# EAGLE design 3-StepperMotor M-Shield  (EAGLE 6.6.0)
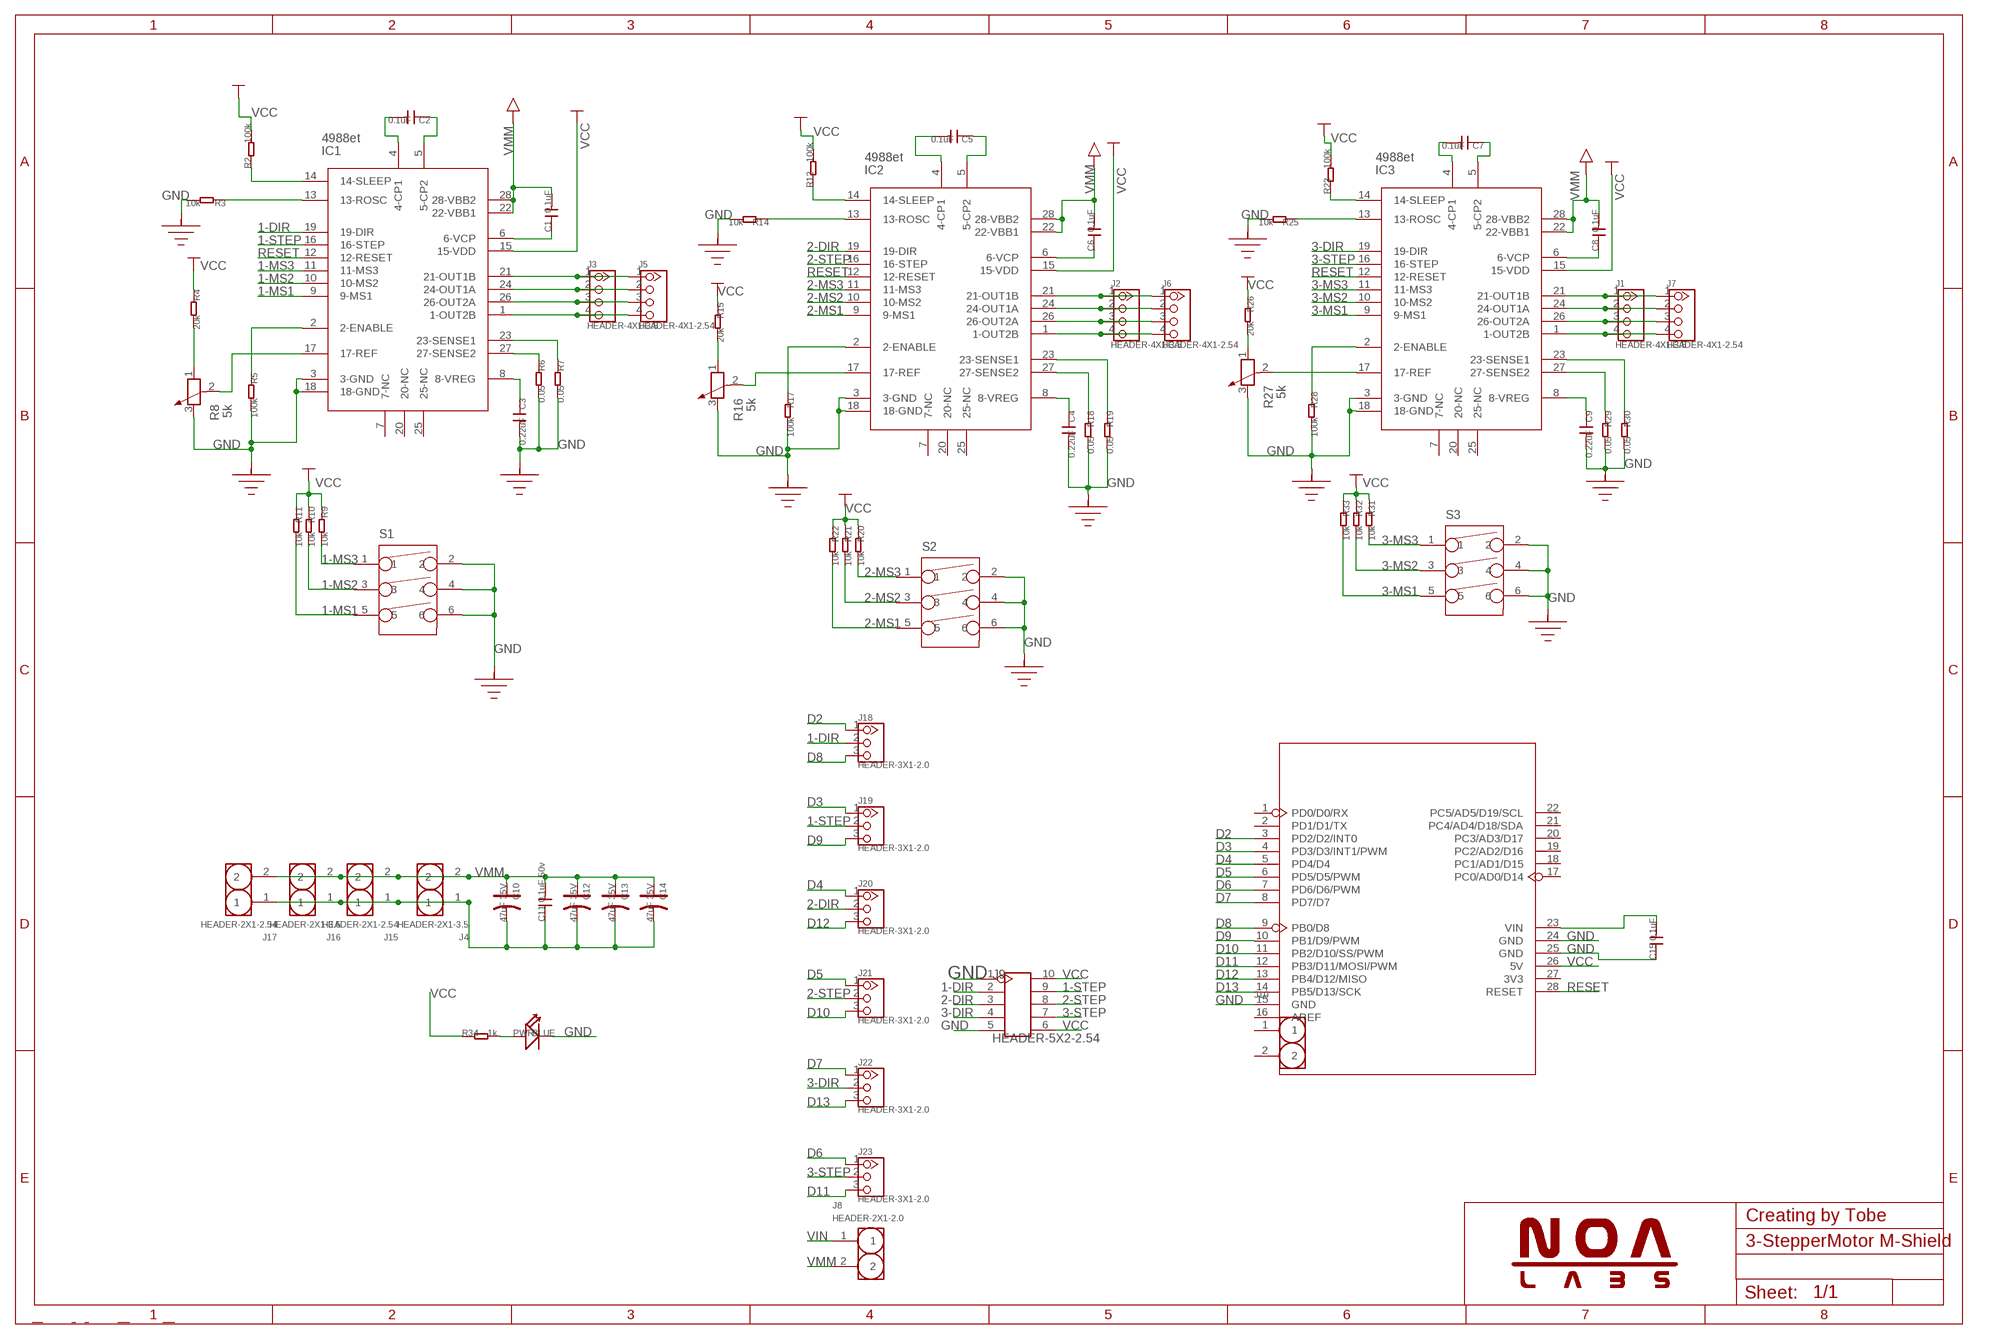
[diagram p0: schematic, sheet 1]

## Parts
C1  0.1uF  C-0603  [0603]
C2  0.1uF  C-0603  [0603]
C3  0.22uF  C-0603  [0603]
C4  0.22uF  C-0603  [0603]
C5  0.1uF  C-0603  [0603]
C6  0.1uF  C-0603  [0603]
C7  0.1uF  C-0603  [0603]
C8  0.1uF  C-0603  [0603]
C9  0.22uF  C-0603  [0603]
C10  47uF 35V  CAP-ELECTRO-E  [ELECTRO-SMD-E-7.8MM]
C11  0.1uF 50v  C-0603  [0603]
C12  47uF 35V  CAP-ELECTRO-E  [ELECTRO-SMD-E-7.8MM]
C13  47uF 35V  CAP-ELECTRO-E  [ELECTRO-SMD-E-7.8MM]
C14  47uF 35V  CAP-ELECTRO-E  [ELECTRO-SMD-E-7.8MM]
C15  0.1uF  C-0603  [0603]
IC1  4988et  A4988Q  [QFN28]
IC2  4988et  A4988Q  [QFN28]
IC3  4988et  A4988Q  [QFN28]
J1  HEADER-4X1-3.5  HEADER-4P3.5  [4P-3.5]
J2  HEADER-4X1-3.5  HEADER-4P3.5  [4P-3.5]
J3  HEADER-4X1-3.5  HEADER-4P3.5  [4P-3.5]
J4  HEADER-2X1-3.5  HEADER-2P3.5  [2P-3.5]
J5  HEADER-4X1-2.54  HEADER-4P-80/40MIL  [4P-2.54-80/40MIL]
J6  HEADER-4X1-2.54  HEADER-4P-80/40MIL  [4P-2.54-80/40MIL]
J7  HEADER-4X1-2.54  HEADER-4P-80/40MIL  [4P-2.54-80/40MIL]
J8  HEADER-2X1-2.0  HEADER-2P-2.0  [2P-2.0]
J9  HEADER-5X2-2.54  HEADER-2X5P-2.54  [2X5P-2.54]
J10  HEADER-2P-65/35MIL  [2P-2.54-65/35MIL]
J15  HEADER-2X1-2.54  HEADER-2P-65/35MIL  [2P-2.54-65/35MIL]
J16  HEADER-2X1-3.5  HEADER-2P3.5  [2P-3.5]
J17  HEADER-2X1-2.54  HEADER-2P-65/35MIL  [2P-2.54-65/35MIL]
J18  HEADER-3X1-2.0  HEADER-3P-2.0  [3P-2.0]
J19  HEADER-3X1-2.0  HEADER-3P-2.0  [3P-2.0]
J20  HEADER-3X1-2.0  HEADER-3P-2.0  [3P-2.0]
J21  HEADER-3X1-2.0  HEADER-3P-2.0  [3P-2.0]
J22  HEADER-3X1-2.0  HEADER-3P-2.0  [3P-2.0]
J23  HEADER-3X1-2.0  HEADER-3P-2.0  [3P-2.0]
PWR  BLUE  LED'0603'  [LED-0603]
R2  100k  R-0603  [0603]
R3  10k  R-0603  [0603]
R4  20k  R-0603  [0603]
R5  100k  R-0603  [0603]
R6  0.05  R-0603  [0603]
R7  0.05  R-0603  [0603]
R8  5k  R-POTENTIOMETER  [3314J]
R9  10k  R-0603  [0603]
R10  10k  R-0603  [0603]
R11  10k  R-0603  [0603]
R12  100k  R-0603  [0603]
R14  10k  R-0603  [0603]
R15  20k  R-0603  [0603]
R16  5k  R-POTENTIOMETER  [3314J]
R17  100k  R-0603  [0603]
R18  0.05  R-0603  [0603]
R19  0.05  R-0603  [0603]
R20  10k  R-0603  [0603]
R21  10k  R-0603  [0603]
R22  10k  R-0603  [0603]
R23  100k  R-0603  [0603]
R25  10k  R-0603  [0603]
R26  20k  R-0603  [0603]
R27  5k  R-POTENTIOMETER  [3314J]
R28  100k  R-0603  [0603]
R29  0.05  R-0603  [0603]
R30  0.05  R-0603  [0603]
R31  10k  R-0603  [0603]
R32  10k  R-0603  [0603]
R33  10k  R-0603  [0603]
R34  1k  R-0603  [0603]
S1  dial switch  DIP-SWITCH-3  [DIP-SWITCH-3]
S2  dial switch  DIP-SWITCH-3  [DIP-SWITCH-3]
S3  dial switch  DIP-SWITCH-3  [DIP-SWITCH-3]
U1  SEEEDUINO-W/O-ISP-HOLE  [SEEEDUINO-W/O-ISP]

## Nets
1-DIR: IC1.19(19-DIR) J9.2 J18.2
1-MS1: IC1.9(9-MS1) R11.2 S1.5
1-MS2: IC1.10(10-MS2) R10.2 S1.3
1-MS3: IC1.11(11-MS3) R9.2 S1.1
1-STEP: IC1.16(16-STEP) J9.9 J19.2
2-DIR: IC2.19(19-DIR) J9.3 J20.2
2-MS1: IC2.9(9-MS1) R22.2 S2.5
2-MS2: IC2.10(10-MS2) R21.2 S2.3
2-MS3: IC2.11(11-MS3) R20.2 S2.1
2-STEP: IC2.16(16-STEP) J9.8 J21.2
3-DIR: IC3.19(19-DIR) J9.4 J22.2
3-MS1: IC3.9(9-MS1) R33.2 S3.5
3-MS2: IC3.10(10-MS2) R32.2 S3.3
3-MS3: IC3.11(11-MS3) R31.2 S3.1
3-STEP: IC3.16(16-STEP) J9.7 J23.2
D2: J18.1 U1.3(PD2/D2/INT0)
D3: J19.1 U1.4(PD3/D3/INT1/PWM)
D4: J20.1 U1.5(PD4/D4)
D5: J21.1 U1.6(PD5/D5/PWM)
D6: J23.1 U1.7(PD6/D6/PWM)
D7: J22.1 U1.8(PD7/D7)
D8: J18.3 U1.9(PB0/D8)
D9: J19.3 U1.10(PB1/D9/PWM)
D10: J21.3 U1.11(PB2/D10/SS/PWM)
D11: J23.3 U1.12(PB3/D11/MOSI/PWM)
D12: J20.3 U1.13(PB4/D12/MISO)
D13: J22.3 U1.14(PB5/D13/SCK)
GND: C3.2 C4.2 C9.2 C10.- C11.1 C12.- C13.- C14.- C15.1 IC1.3(3-GND) IC1.18(18-GND) IC2.3(3-GND) IC2.18(18-GND) IC3.3(3-GND) IC3.18(18-GND) J4.1 J9.1 J9.5 J15.1 J16.1 J17.1 PWR.- R3.2 R5.2 R6.2 R7.2 R8.3 R14.2 R16.3 R17.2 R18.2 R19.2 R25.2 R27.3 R28.2 R29.2 R30.2 S1.2 S1.4 S1.6 S2.2 S2.4 S2.6 S3.2 S3.4 S3.6 U1.15(GND) U1.24(GND) U1.25(GND) ; supply symbol labelled GND_POWER
N$1: IC1.14(14-SLEEP) R2.1
N$2: IC1.17(17-REF) R8.2
N$3: IC2.14(14-SLEEP) R12.1
N$4: IC1.13(13-ROSC) R3.1
N$5: IC1.2(2-ENABLE) R5.1
N$6: IC1.27(27-SENSE2) R6.1
N$7: IC1.23(23-SENSE1) R7.1
N$8: C3.1 IC1.8(8-VREG)
N$9: C1.1 IC1.6(6-VCP)
N$10: IC2.13(13-ROSC) R14.1
N$11: IC3.14(14-SLEEP) R23.1
N$12: C2.1 IC1.5(5-CP2)
N$13: C2.2 IC1.4(4-CP1)
N$14: IC3.13(13-ROSC) R25.1
N$15: IC1.21(21-OUT1B) J3.1 J5.1
N$16: IC1.24(24-OUT1A) J3.2 J5.2
N$17: IC1.26(26-OUT2A) J3.3 J5.3
N$18: IC1.1(1-OUT2B) J3.4 J5.4
N$19: IC2.17(17-REF) R16.2
N$20: R4.2 R8.1
N$21: R15.2 R16.1
N$22: PWR.+ R34.2
N$23: R26.2 R27.1
N$28: IC2.2(2-ENABLE) R17.1
N$30: IC2.27(27-SENSE2) R18.1
N$31: C4.1 IC2.8(8-VREG)
N$32: IC2.23(23-SENSE1) R19.1
N$34: IC2.1(1-OUT2B) J2.4 J6.4
N$35: IC2.26(26-OUT2A) J2.3 J6.3
N$36: IC2.24(24-OUT1A) J2.2 J6.2
N$37: IC2.21(21-OUT1B) J2.1 J6.1
N$38: C6.1 IC2.6(6-VCP)
N$39: IC3.2(2-ENABLE) R28.1
N$40: IC3.17(17-REF) R27.2
N$41: C5.1 IC2.5(5-CP2)
N$42: C5.2 IC2.4(4-CP1)
N$45: C9.1 IC3.8(8-VREG)
N$46: IC3.27(27-SENSE2) R29.1
N$47: IC3.23(23-SENSE1) R30.1
N$48: C8.1 IC3.6(6-VCP)
N$50: C7.1 IC3.5(5-CP2)
N$51: C7.2 IC3.4(4-CP1)
N$59: IC3.21(21-OUT1B) J1.1 J7.1
N$60: IC3.24(24-OUT1A) J1.2 J7.2
N$61: IC3.26(26-OUT2A) J1.3 J7.3
N$62: IC3.1(1-OUT2B) J1.4 J7.4
RESET: IC1.12(12-RESET) IC2.12(12-RESET) IC3.12(12-RESET) U1.28(RESET)
VCC: IC1.15(15-VDD) IC2.15(15-VDD) IC3.15(15-VDD) J9.6 J9.10 R2.2 R4.1 R9.1 R10.1 R11.1 R12.2 R15.1 R20.1 R21.1 R22.1 R23.2 R26.1 R31.1 R32.1 R33.1 R34.1 U1.26(5V) ; supply symbol labelled POWER_BAR
VIN: C15.2 J8.1 U1.23(VIN)
VMM: C1.2 C6.2 C8.2 C10.+ C11.2 C12.+ C13.+ C14.+ IC1.22(22-VBB1) IC1.28(28-VBB2) IC2.22(22-VBB1) IC2.28(28-VBB2) IC3.22(22-VBB1) IC3.28(28-VBB2) J4.2 J8.2 J15.2 J16.2 J17.2 ; supply symbol labelled POWER_ARROW
Unconnected: IC1.7(7-NC) IC1.20(20-NC) IC1.25(25-NC) IC2.7(7-NC) IC2.20(20-NC) IC2.25(25-NC) IC3.7(7-NC) IC3.20(20-NC) IC3.25(25-NC) J10.1 J10.2 U1.1(PD0/D0/RX) U1.2(PD1/D1/TX) U1.16(AREF) U1.17(PC0/AD0/D14) U1.18(PC1/AD1/D15) U1.19(PC2/AD2/D16) U1.20(PC3/AD3/D17) U1.21(PC4/AD4/D18/SDA) U1.22(PC5/AD5/D19/SCL) U1.27(3V3)

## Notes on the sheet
- Creating by Tobe

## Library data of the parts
C1-C9 C11 C15 = Discrete:C*: Ceramic Capacitors
C10 C12-C14 = Discrete:CAP*: Electrolytic Capacitors,Tantalum Capacitors and Super Capacitors
IC1-IC3 = IC:A4988
J1-J3 J5-J7 = Connector:HEADER-4P
J4 J8 J10 J15-J17 = Connector:HEADER-2P
J9 = Connector:HEADER-2X5P
J18-J23 = Connector:HEADER-3P
PWR = Discrete:LED*
R2-R7 R9-R12 R14 R15 R17-R23 R25 R26 R28-R34 = Discrete:R*
R8 R16 R27 = Discrete:R-POTENTIOMETER*: Potentiometer
S1-S3 = Discrete:DIP-SWITCH-3
U1 = Module:SEEEDUINO-W/O-ISP

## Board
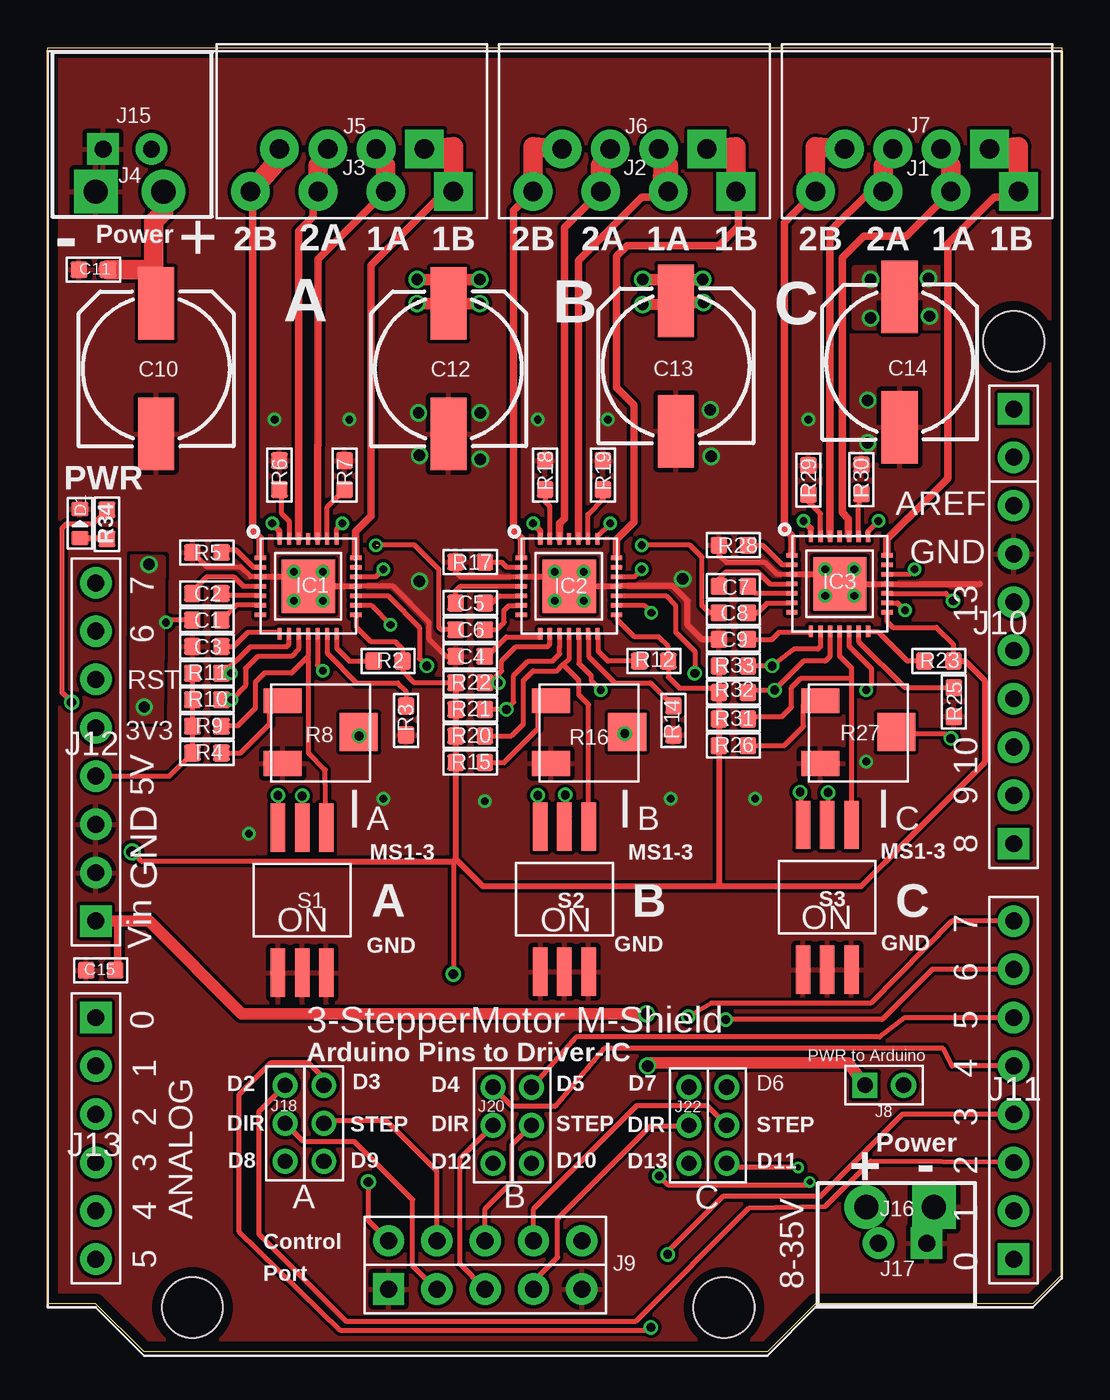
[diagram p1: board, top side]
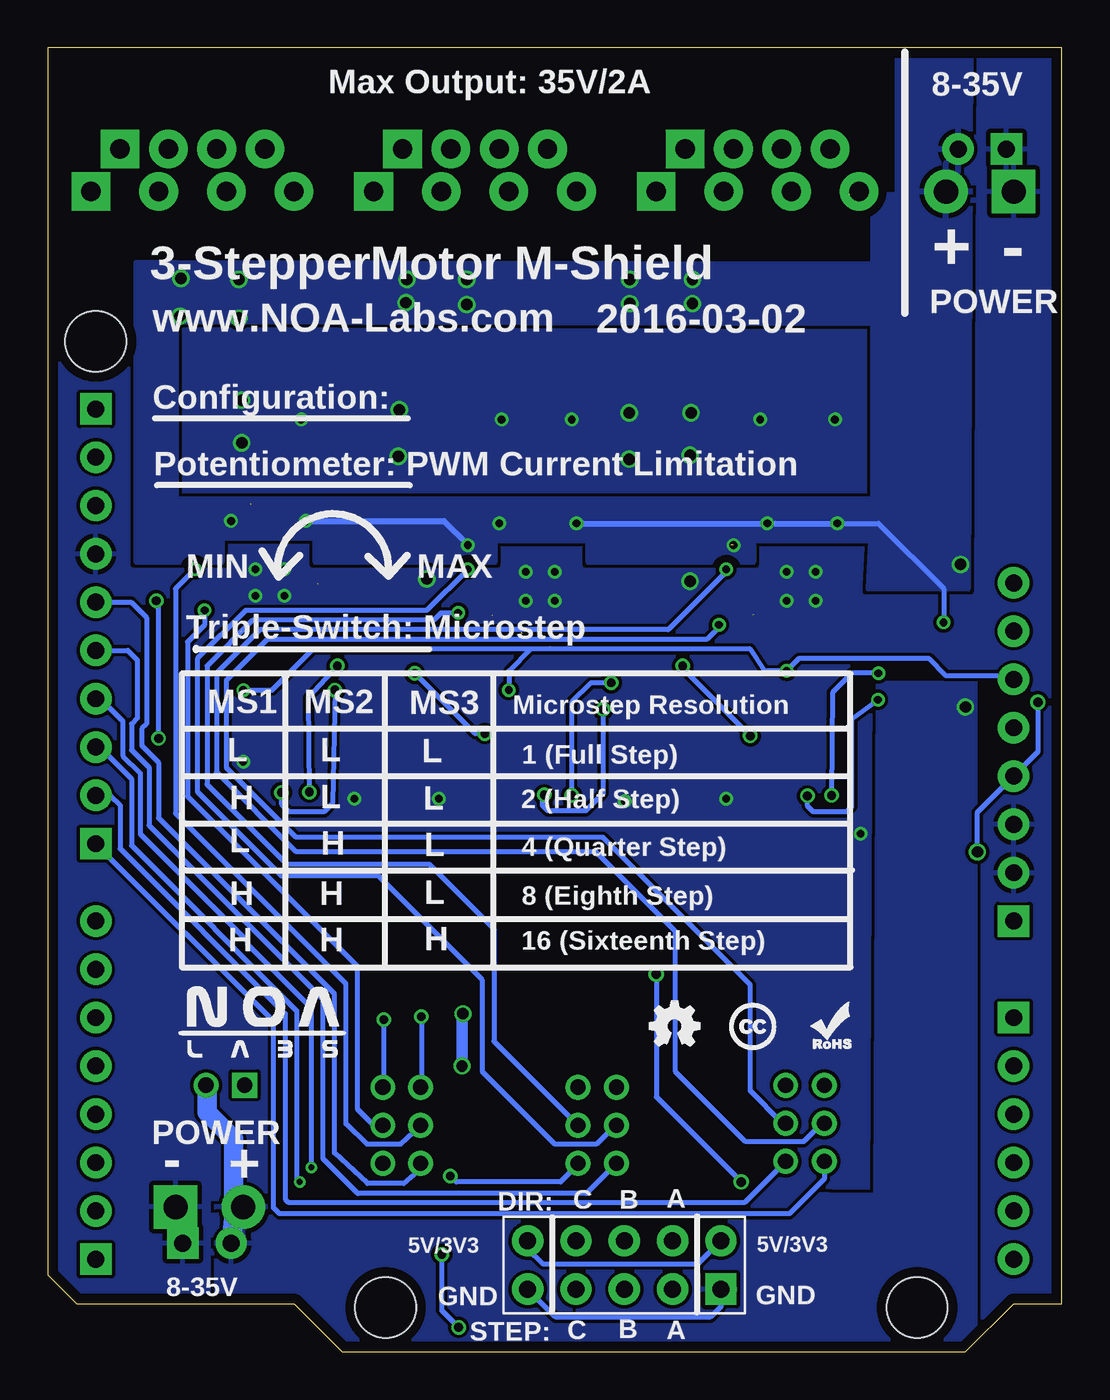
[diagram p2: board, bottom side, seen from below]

Size 53.34 x 68.58 mm. Coordinates in mm from the lower left corner, seen from the top.
Outline: 0,68.58 53.34,68.58 53.34,4.06 51.82,2.54 40.39,2.54 37.85,0 5.08,0 2.54,2.54 0,2.54 0,68.58
Copper layers (1*16): Top 0.035mm / dielectric 1.5mm / Bottom 0.035mm
Design rules "NOA Eagle Rule": minimum track width 7mil, minimum drill 12mil, track to track 7mil, track to pad 7mil, pad to pad 7mil, via to via 7mil, smd to smd 0mil, copper to edge 20mil, drill to drill 10mil, minimum pad ring 10mil, minimum via ring 6mil, stop-mask expansion 2mil, vias tented up to drill 25mil, thermal gap 10mil

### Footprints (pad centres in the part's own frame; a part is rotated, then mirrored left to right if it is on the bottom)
0603 = smd 0.889 x 0.889: 1 -0.762,0; 2 0.762,0
ELECTRO-SMD-E-7.8MM = smd 3.81 x 1.905: + 3.429,0; - -3.429,0
QFN28 = smd 0.6 x 0.23: 1 -2.516,1.5; 2 -2.516,1; 3 -2.516,0.5; 4 -2.516,0; 5 -2.516,-0.5; 6 -2.516,-1; 7 -2.516,-1.5; 15 2.484,-1.5; 16 2.484,-1; 17 2.484,-0.5; 18 2.484,0; 19 2.484,0.5; 20 2.484,1; 21 2.484,1.5 | smd 0.23 x 0.6: 8 -1.516,-2.5; 9 -1.016,-2.5; 10 -0.516,-2.5; 11 -0.016,-2.5; 12 0.484,-2.5; 13 0.984,-2.5; 14 1.484,-2.5; 22 1.484,2.5; 23 0.984,2.5; 24 0.484,2.5; 25 -0.016,2.5; 26 -0.516,2.5; 27 -1.016,2.5; 28 -1.516,2.5 | smd 2.8 x 2.8: 29 0,0
4P-3.5 = drill 1.016 pad 2.032 square: 1 0,5.334 | drill 1.016 pad 2.032: 2 0,1.778; 3 0,-1.778; 4 0,-5.334
2P-3.5 = drill 1.27 pad 2.286 square: 1 0,-1.651 | drill 1.27 pad 2.286: 2 0,1.905
4P-2.54-80/40MIL = drill 1.016 pad 2.032 square: 1 0,3.81 | drill 1.016 pad 2.032: 2 0,1.27; 3 0,-1.27; 4 0,-3.81
2P-2.0 = drill 0.813 pad 1.27 square: 1 -1.016,0 | drill 0.813 pad 1.27: 2 1.016,0
2X5P-2.54 = drill 0.889 pad 1.651 square: 1 -1.27,5.08 | drill 0.889 pad 1.651: 2 -1.27,2.54; 3 -1.27,0; 4 -1.27,-2.54; 5 -1.27,-5.08; 6 1.27,-5.08; 7 1.27,-2.54; 8 1.27,0; 9 1.27,2.54; 10 1.27,5.08
2P-2.54-65/35MIL = drill 0.889 pad 1.651 square: 1 0,1.27 | drill 0.889 pad 1.651: 2 0,-1.27
3P-2.0 = drill 0.8: 1 0,0; 2 2,0; 3 4,0
LED-0603 = smd 0.762 x 0.889: + -0.762,0; - 0.762,0
3314J = smd 1.3 x 2: 1 1.65,4; 3 -1.65,4 | smd 2 x 2: 2 0,0
DIP-SWITCH-3 = smd 2.54 x 0.762: 1 -6.985,0.635; 2 0.635,0.635; 3 -6.985,-0.635; 4 0.635,-0.635; 5 -6.985,-1.905; 6 0.635,-1.905
SEEEDUINO-W/O-ISP = drill 0.889 pad 1.651 square: 1 63.5,50.8; 9 41.656,50.8; 17 50.8,2.54; 23 45.72,2.54 | drill 0.889 pad 1.651: 2 60.96,50.8; 3 58.42,50.8; 4 55.88,50.8; 5 53.34,50.8; 6 50.8,50.8; 7 48.26,50.8; 8 45.72,50.8; 10 39.116,50.8; 11 36.576,50.8; 12 34.036,50.8; 13 31.496,50.8; 14 28.956,50.8; 15 26.416,50.8; 16 23.876,50.8; 18 53.34,2.54; 19 55.88,2.54; 20 58.42,2.54; 21 60.96,2.54; 22 63.5,2.54; 24 43.18,2.54; 25 40.64,2.54; 26 38.1,2.54; 27 35.56,2.54; 28 33.02,2.54; 29 30.48,2.54; 30 27.94,2.54 | hole 3.2: 15.24,50.8; 66.04,35.56; 66.04,7.62

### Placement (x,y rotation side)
C1  8.38,38.48 180 top
C2  8.38,39.88 180 top
C3  8.38,37.08 180 top
C4  22.23,36.58 180 top
C5  22.23,39.37 180 top
C6  22.23,37.97 180 top
C7  36.07,40.26 180 top
C8  36.07,38.86 180 top
C9  36.07,37.46 180 top
C10  5.71,51.69 90 top
C11  2.41,56.9 0 top
C12  21.08,51.69 90 top
C13  33.05,51.84 90 top
C14  44.81,52.04 90 top
C15  2.79,20.07 0 top
IC1  13.72,40.26 0 top
IC2  27.43,40.26 0 top
IC3  41.66,40.39 0 top
J1  45.72,61.01 270 top
J2  30.86,61.01 270 top
J3  16,61.01 270 top
J4  4.19,61.01 270 top
J5  16,63.25 270 top
J6  30.86,63.25 270 top
J7  45.72,63.25 270 top
J8  43.99,14.02 0 top
J9  23.01,4.57 90 top
J10  50.8,48.31 0 top
J15  4.19,63.25 90 top
J16  44.96,7.62 90 top
J17  44.96,5.71 270 top
J18  12.5,14.02 270 top
J19  14.53,14.02 270 top
J20  23.42,13.92 270 top
J21  25.45,13.92 270 top
J22  33.73,13.92 270 top
J23  35.71,13.92 270 top
PWR  1.7,43.56 90 top
R2  17.91,36.32 0 top
R3  18.85,33.2 270 top
R4  8.38,31.5 0 top
R5  8.38,42.04 180 top
R6  12.19,46.1 90 top
R7  15.62,46.1 90 top
R8  16.36,32.59 90 top
R9  8.38,32.89 0 top
R10  8.38,34.29 0 top
R11  8.38,35.69 0 top
R12  31.88,36.32 0 top
R14  32.92,33.2 270 top
R15  22.23,30.99 0 top
R16  30.48,32.59 90 top
R17  22.23,41.53 180 top
R18  26.16,46.1 90 top
R19  29.21,46.1 90 top
R20  22.23,32.38 0 top
R21  22.23,33.78 0 top
R22  22.23,35.18 0 top
R23  46.86,36.32 0 top
R25  47.65,34.16 270 top
R26  36.07,31.88 0 top
R27  44.63,32.59 90 top
R28  36.07,42.42 180 top
R29  40.01,45.85 90 top
R30  42.8,45.87 90 top
R31  36.07,33.27 0 top
R32  36.07,34.67 0 top
R33  36.07,36.07 0 top
R34  3.12,43.51 270 top
S1  14.02,20.57 270 top
S2  27.81,20.62 270 top
S3  41.63,20.73 270 top
U1  0,68.38 270 top

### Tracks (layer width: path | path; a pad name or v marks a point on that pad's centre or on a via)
1-DIR  (via drill 0.41)
  Top 0.254: IC1.19 17.26,40.76 v17.65,41.15 | J9.2 20.42,3.3 19.2,4.52 19.2,8 16.15,11.05 13.47,11.05 J18.2
  Bottom 0.254: v17.65,41.15 17.65,41.02 20.7,37.97 42.16,37.97 44.45,35.69 44.45,30.48 40.26,26.29 24.51,26.29 20.32,22.1 20.32,14.73 16.64,11.05 13.59,11.05 12.62,12.02 J18.2
1-MS1  (via drill 0.41, 0.46)
  Top 0.254: R11.2 9.27,35.69 | 9.27,35.69 10.67,37.08 12.57,37.08 12.7,37.21 IC1.9 | 9.27,35.69 v9.65,35.69 | v12.12,29.26 S1.5
  Bottom 0.254: v9.65,35.69 11.05,35.69 12.06,34.67 v12.12,29.26
1-MS2  (via drill 0.41, 0.46)
  Top 0.254: IC1.10 13.2,36.95 12.83,36.58 11.05,36.58 10.41,35.94 10.41,35.03 v9.68,34.29 R10.2 | S1.3 v13.39,29.23
  Bottom 0.254: v9.68,34.29 11.05,33.27 11.05,28.68 11.33,28.4 13.08,28.4 13.39,28.7 v13.39,29.23
1-MS3
  Top 0.254: IC1.11 13.7,36.56 13.65,36.51 | 13.65,36.51 12.83,35.69 11.4,35.69 10.92,35.2 10.92,33.83 10.01,32.92 9.17,32.92 R9.2 | S1.1 14.61,30.61 13.72,31.5 13.72,36.45 13.65,36.51
1-STEP  (via drill 0.41)
  Top 0.254: IC1.16 17,39.26 v18.03,38.23 | J9.9 20.47,9.5 17.83,12.14 14.65,12.14 J19.2
  Bottom 0.254: v18.03,38.23 18.03,38.1 18.67,37.46 41.78,37.46 43.94,35.31 43.94,30.73 40.26,27.05 24.13,27.05 16.38,19.3 16.38,13.72 14.69,12.02 J19.2
2-DIR  (via drill 0.41)
  Top 0.254: IC2.19 30.85,40.76 v31.24,41.15 | J9.3 21.69,4.62 21.69,10.19 J20.2
  Bottom 0.254: v31.24,41.15 33.4,38.99 42.93,38.99 45.47,36.45 45.47,29.46 41.02,25.02 35.94,25.02 30.48,19.56 30.48,14.73 26.67,10.92 24.49,10.92 23.49,11.92 J20.2
2-MS1  (via drill 0.46)
  Top 0.254: R22.2 23.24,35.18 23.5,35.43 | 23.5,35.43 23.88,35.81 23.88,36.32 24.64,37.08 26.29,37.08 26.42,37.21 IC2.9 | 23.5,35.43 23.62,35.43 v23.7,35.18 | v25.78,29.26 25.78,28.45 S2.5
  Bottom 0.254: v23.7,35.18 24.77,35.18 25.78,34.16 v25.78,29.26
2-MS2  (via drill 0.46)  (1 unrouted)
  Top 0.254: IC2.10 26.92,37.08 | R21.2 v24.13,33.78 24.51,34.16 24.51,35.56 25.27,36.32 26.54,36.32 26.92,36.7 26.92,37.08 | v27.23,29.29 27.43,28.07 S2.3
  Bottom 0.254: v24.13,33.78 24.13,29.36 25.04,28.45 27.04,28.45 27.32,28.73 27.32,29.19 v27.23,29.29
2-MS3
  Top 0.254: R20.2 24.38,32.38 25.02,33.02 25.02,35.31 25.53,35.81 26.8,35.81 27.11,36.13 | 27.11,36.13 27.43,36.45 27.43,37.74 IC2.11 | 27.11,36.13 27.94,35.31 27.94,34.54 28.45,34.04 S2.1
2-STEP  (via drill 0.41)
  Top 0.254: IC2.16 31.35,39.26 v31.75,38.86 | J9.8 23.01,7.52 24.43,8.94 24.43,10.9 J21.2
  Bottom 0.254: v31.75,38.86 32.64,38.86 33.02,38.48 42.55,38.48 44.96,36.07 44.96,29.84 40.77,25.65 33.27,25.65 29.87,22.25 29.87,16.34 J21.2
3-DIR  (via drill 0.41)
  Top 0.254: IC3.19 45.33,40.89 v45.59,41.15 | J9.4 25.55,3.71 26.82,4.98 26.82,7.01 31.7,11.89 33.7,11.89 J22.2
  Bottom 0.254: v45.59,41.15 46.61,40.13 46.61,28.32 37.64,19.36 37.64,11.99 36.55,10.92 34.77,10.92 33.73,11.89 J22.2
3-MS1  (via drill 0.46)
  Top 0.254: v39.57,29.44 S3.5 | R33.2 v38.1,36.07 39.24,36.96 40.51,36.96 40.64,37.08 IC3.9
  Bottom 0.254: v39.57,29.44 39.62,34.42 v38.1,36.07
3-MS2  (via drill 0.46)
  Top 0.254: IC3.10 41.15,37.88 41.15,36.58 40.89,36.32 39.75,36.32 v38.23,34.8 36.96,34.8 R32.2 | S3.3 v41.05,29.41
  Bottom 0.254: v38.23,34.8 38.35,28.85 38.81,28.4 40.64,28.4 41.03,28.79 41.03,29.39 v41.05,29.41
3-MS3
  Top 0.254: IC3.11 41.66,37.87 41.66,36.58 42.27,35.97 42.27,35.43 | R31.2 36.96,33.4 38.61,33.4 39.12,33.91 39.12,34.92 39.62,35.43 42.27,35.43 | 42.27,35.43 S3.1
3-STEP  (via drill 0.41)
  Top 0.254: IC3.16 44.69,39.39 v45.09,38.99 | J9.7 25.55,7.52 30.99,12.95 34.68,12.95 J23.2
  Bottom 0.254: v45.09,38.99 45.09,38.23 45.97,37.34 45.97,29.21 37.03,20.27 37.03,12.75 36.2,11.92 J23.2
D2
  Top 0.254: U1.3 43.28,10.03 40.89,7.65 36.88,7.57 30.94,1.63 15.7,1.63 11.12,6.2 11.12,12.65 J18.1
D3  (via drill 0.46)
  Top 0.254: U1.4 44.96,12.5 40.64,8.18 35.51,8.18 35.48,8.15 32.61,5.28 v32.61,5.13 | J19.1 14.53,14.38 13.72,15.19 11.73,15.19 10.06,13.51 10.06,6.35 15.39,1.14 31.7,1.14 v31.73,1.29
  Bottom 0.254: v32.61,5.13 32.61,2.18 v31.73,1.29
D4
  Top 0.254: U1.5 47.55,15.04 47.09,15.95 29.26,15.95 26.67,12.9 24.43,12.9 J20.1
D5
  Top 0.254: U1.6 45.06,17.58 43.74,16.56 27.79,16.56 J21.1
D6  (via drill 0.46)
  Top 0.254: U1.7 46.53,20.12 43.89,17.48 v35.66,17.48
  Bottom 0.254: v35.66,17.48 35.66,13.97 J23.1
D7  (via drill 0.46)
  Top 0.254: U1.8 47.55,22.66 43.28,18.34 34.9,18.34 v33.68,17.63
  Bottom 0.254: v33.68,17.63 33.68,13.97 J22.1
D8
  Bottom 0.254: J18.3 12.5,9.09 14.33,7.26 41.15,7.26 41.45,7.57 41.45,17.37 U1.9
D9
  Bottom 0.254: U1.10 50.04,29.26 49.53,28.75 49.53,26.47 40.84,17.78 40.84,8.03 40.69,7.87 16.68,7.87 J19.3
D10  (via drill 0.3, 0.46)
  Top 0.254: v32.16,9.25 32.61,8.79 39.93,8.79 v40.08,8.94
  Bottom 0.254: U1.11 50.6,31.8 48.92,30.12 48.92,26.62 40.23,17.93 40.23,9.09 v40.08,8.94 | J21.3 25.45,9.86 26.36,8.94 31.85,8.94 v32.16,9.25
D11  (via drill 0.3)
  Top 0.254: 35.78,9.86 J23.3 | J23.3 35.75,9.92 36.12,9.55 | v39.47,9.7 35.93,9.7 J23.3
  Bottom 0.254: U1.12 50.55,34.34 49.38,33.17 49.38,31.34 48.46,30.43 48.46,27.23 42.82,21.59 42.82,21.44 39.47,18.09 v39.47,9.7
D12
  Bottom 0.254: U1.13 49.12,36.88 48.62,36.37 48.62,33.33 48.92,33.02 48.92,31.65 48.01,30.73 48.01,27.69 38.86,18.54 38.86,10.16 37.03,8.33 25.01,8.33 J20.3
D13
  Bottom 0.254: U1.14 48.95,39.42 48.13,38.61 48.13,33.02 48.39,32.77 48.39,31.88 47.5,30.99 47.5,28.07 38.25,18.82 38.25,10.46 36.52,8.87 34.59,8.87 33.73,9.6 J22.3
GND  (via drill 0.41, 0.6)
  Top 0.254: R17.2 21.46,41.02 21.72,40.77 24.91,40.77 IC2.3 | IC1.3 10.68,40.76 10.16,41.27 8.38,41.27 R5.2 | R28.2 35.31,41.91 35.69,41.53 37.72,41.53 38.35,40.89 IC3.3 | C4.2 20.95,36.58 20.07,37.46 20.07,38.35 18.16,40.26 IC1.18 | 27.19,40.76 26.93,40.76 v26.67,41.02 | 42.16,40.39 42.16,40.01 v42.42,39.75 | 14.22,40.26 14.22,39.75 v14.48,39.5
  Top 0.305: IC1.3 13.72,40.76 14.22,40.26 IC1.18 | IC2.3 27.19,40.76 27.69,40.26 IC2.18 32.89,40.26 33.66,39.5 33.66,38.23 34.42,37.46 C9.2 | IC3.3 41.66,40.89 42.16,40.39 IC3.18 49.02,40.39
  Bottom 0.254: J9.1 17.93,2.39 18.49,1.83 26.62,1.83 J9.5
  other vias: 12.95,41.02 12.95,39.5 14.48,41.02 26.67,39.5 28.19,41.02 28.19,39.5 40.89,41.15 42.42,41.15 40.89,39.75 11.94,49.02 15.88,49.02 25.78,49.02 29.46,49.02 40.01,49.02 17.65,29.08 22.99,28.96 32.77,29.08 37.21,29.08 19.51,49.38 19.56,47.14 22.76,49.38 22.76,46.94 34.85,49.53 34.9,47.09 43.13,50.04 43.13,47.8 33.4,40.64 19.56,40.51 43.05,31.04 10.59,27.25
  pour Bottom (rank 2): -0.13,68.71 53.34,68.71 53.34,-0.13 -0.13,-0.13
  pour Top (rank 2): -0.13,68.71 53.34,68.71 53.34,-0.13 -0.13,-0.13
N$1
  Top 0.254: IC1.14 15.2,37 15.88,36.32 R2.1
N$2  (via drill 0.46)
  Top 0.254: v16.38,32.38 15.93,32.38 R8.2 | v19.94,36.07 19.56,36.45 19.56,38.1 17.9,39.76 IC1.17
  Bottom 0.254: v16.38,32.38 19.68,35.69 19.68,35.81 v19.94,36.07
N$3
  Top 0.254: R12.1 29.46,36.32 28.96,36.83 28.96,37.72 IC2.14
N$4
  Top 0.254: IC1.13 14.7,36.73 16.26,35.18 18.41,35.18 18.85,34.75 R3.1
N$5
  Top 0.254: IC1.2 10.81,41.26 9.91,42.16 9.27,42.16 R5.1
N$6
  Top 0.254: R6.1 12.32,45.21 12.32,44.07 12.7,43.69 IC1.27
N$7
  Top 0.254: IC1.23 14.7,44.42 R7.1
N$8
  Top 0.254: C3.1 9.78,37.08 10.54,37.85 12.11,37.85 IC1.8
N$9
  Top 0.254: IC1.6 9.92,39.26 C1.1
N$10  (1 unrouted)
  Top 0.254: 28.45,37.85 28.45,36.58 29.84,35.18 31.7,35.18 R14.1
N$11  (1 unrouted)
  Top 0.254: R23.1 45.21,36.32 43.69,37.85 43.18,37.85
N$12
  Top 0.254: IC1.5 9.26,39.76 C2.1
N$13
  Top 0.254: C2.2 7.62,40.01 8.38,40.77 9.78,40.77 10.29,40.26 IC1.4
N$14
  Top 0.254: IC3.13 42.67,37.85 42.67,37.34 45.09,34.92 R25.1
N$15
  Top 0.406: IC1.21 16.2,43.12 17.02,43.94 17.02,57.15 20.57,60.71 21.03,60.71 J3.1
  Top 1.016: J3.1 21.34,63.37 J5.1
N$16
  Top 0.406: IC1.24 14.2,44.22 14.2,47.68 14.22,47.68 14.22,57.45 J3.2
  Top 1.016: J3.2 17.78,62.36 J5.2
N$17
  Top 0.406: IC1.26 13.2,58.92 13.97,59.69 13.97,60.76 J3.3
  Top 1.016: J3.3 14.22,62.36 J5.3
N$18  (1 unrouted)
  Top 0.254: 11.18,41.91 11.2,41.91 IC1.1
  Top 0.406: 11.2,60.86 J5.4 | 11.18,60.83 10.79,60.45 10.79,43.18 11.2,42.77 11.18,42.77 11.18,41.91
  Top 1.016: J5.4 12.19,62.74 J3.4
N$19  (via drill 0.46)
  Top 0.254: IC2.17 32.5,39.76 33.02,39.24 33.02,37.85 34.04,36.83 v34.04,35.69 | 29.59,32.38 30.23,32.38 v30.35,32.51
  Top 0.406: v30.35,32.51 30.48,32.51 R16.2
  Bottom 0.254: v30.35,32.51 30.86,32.51 v34.04,35.69
N$20
  Top 0.254: R4.2 10.16,31.5 11.68,33.02 11.68,33.56 R8.1
N$21
  Top 0.254: R15.2 24,30.99 25.78,32.77 25.78,33.74 R16.1
N$22
  Top 0.305: PWR.+ 3.07,42.8 R34.2
N$23
  Top 0.254: R26.2 38.73,31.88 39.75,32.89 39.75,34.04 39.88,34.16 40.55,34.16 R27.1
N$28
  Top 0.254: R17.1 23.88,41.53 24.13,41.27 24.9,41.27 IC2.2
N$30
  Top 0.254: IC2.27 26.42,44.45 26.16,44.7 R18.1
N$31
  Top 0.254: C4.1 23.11,36.58 24.13,37.59 25.75,37.59 IC2.8
N$32
  Top 0.254: IC2.23 28.42,44.04 29.21,44.83 R19.1
N$34
  Top 0.406: J2.4 24.51,59.99 24.51,43.18 24.92,42.77 IC2.1
  Top 1.016: J2.4 25.53,63.37 J6.4
N$35
  Top 0.406: IC2.26 26.92,43.55 27.18,43.81 27.18,59.11 J2.3 | 29.34,61.59 J6.3
  Top 1.016: J2.3 29.08,62.36 J6.3
N$36
  Top 0.406: IC2.24 27.92,57.38 31.24,60.71 32.33,60.71 J2.2 | 32.26,61.72 J6.2 32,61.72 32,61.01
  Top 1.016: J2.2 32.64,62.36 J6.2
N$37
  Top 0.406: IC2.21 29.92,42.72 30.84,43.64 30.84,49.78 29.92,50.7 29.92,57.61 30.48,58.17 35.31,58.17 36.32,59.18 36.32,60.88 J2.1
  Top 1.016: J2.1 36.2,63.37 J6.1
N$38
  Top 0.254: C6.1 23.62,37.97 24,38.35 24,38.99 24.26,39.24 24.9,39.24 IC2.6
N$39
  Top 0.254: R28.1 37.59,42.42 38.61,41.4 39.12,41.4 IC3.2
N$40  (via drill 0.46)
  Top 0.254: R27.2 44.38,32.51 47.24,32.51 v47.5,32.26 | IC3.17 47.24,39.89 v47.62,39.5
  Bottom 0.254: v47.5,32.26 47.5,39.37 v47.62,39.5
N$41
  Top 0.254: C5.1 23.37,39.37 23.75,39.75 24.91,39.75 IC2.5
N$42
  Top 0.254: C5.2 21.46,40.01 21.72,40.26 IC2.4
N$45
  Top 0.254: C9.1 38.1,37.46 38.48,37.85 40.1,37.85 IC3.8
N$46
  Top 0.254: IC3.27 40.64,44.07 40.01,44.7 R29.1
N$47  (1 unrouted)
  Top 0.254: IC3.23 42.64,44.55 | R30.1 42.72,45.09 42.67,44.58
N$48
  Top 0.254: C8.1 37.34,38.86 37.85,39.37 39.12,39.37 IC3.6
N$50
  Top 0.254: IC3.5 37.2,39.89 C7.1
N$51  (1 unrouted)
  Top 0.254: C7.2 35.31,40.64 35.69,41.02 37.34,41.02 37.97,40.39 39.12,40.39
N$59
  Top 0.406: IC3.21 44.14,42.74 45.21,43.81 45.24,43.81 47.35,45.92 47.35,58.27 49.78,60.71 50.75,60.71 J1.1
  Top 1.016: J1.1 51.05,63.37 J7.1
N$60
  Top 0.406: IC3.24 42.11,42.91 42.11,43.79 41.78,44.12 41.78,57.53 42.93,58.67 45.16,58.67 J1.2
  Top 1.016: J1.2 47.5,62.36 J7.2
N$61
  Top 0.406: IC3.26 41.14,58.92 43.18,60.96 43.89,60.96 J1.3
  Top 1.016: J1.3 43.94,62.36 J7.3
N$62
  Top 0.406: IC3.1 39.14,42.9 38.73,43.31 38.73,59.36 J1.4
  Top 1.016: J1.4 40.39,63.37 J7.4
RESET  (via drill 0.41)
  Top 0.254: IC1.12 14.2,36.09 v14.48,35.81 | IC2.12 27.94,37.73 27.94,36.2 28.57,35.56 28.57,35.31 v29.08,34.8 | IC3.12 42.14,37.11 43.31,35.94 43.31,35.05 v43.05,34.8
  Bottom 0.254: 27.94,36.96 16.38,36.96 15.62,35.81 v14.48,35.81 13.84,36.45 6.99,36.45 6.1,35.56 2.74,35.56 U1.28 | v43.05,34.8 41.53,34.8 39.37,36.96 27.94,36.96 | 27.94,36.96 29.08,35.81 v29.08,34.8
VCC  (via drill 0.5, 0.6)  (2 unrouted)
  Top 0.254: R15.1 R20.1 R21.1 R22.1 21.44,35.2 19.25,35.2 18.67,35.79 R2.2 18.67,36.96 18.29,37.34 17.02,37.34 16.26,38.1 16.26,38.73 | 29.94,38.73 IC2.15 | R23.2 47.62,37.21 46.74,38.1 44.45,38.1 44.14,38.41 IC3.15 | R11.1 R10.1 R9.1 R4.1 6.4,30.28 U1.26 | R26.1 R31.1 R32.1 35.08,34.9 33.22,34.9 32.64,35.48 R12.2 32.64,37.08 32.13,37.59 30.86,37.59 29.97,38.48 29.97,38.73 | 3.05,44.35 R34.1 2.41,43.56 1.02,43.56 0.76,43.31 0.76,34.67 v1.27,34.16 | 21.34,25.78 v21.34,19.86 | v16.87,8.94 16.87,6.91 J9.10 | 11.05,25.78 4.95,25.78 v4.45,26.29 | 44.07,25.78 42.77,24.49 | 35.31,24.54 35.26,24.49
  Top 0.305: 11.05,25.78 21.34,25.78 21.46,25.91 | R22.1 21.46,25.91 | R33.1 R32.1 35.31,24.54 | 44.07,25.78 49.28,30.99 49.28,35.31 48.26,36.32 R23.2 | 42.77,24.49 35.26,24.49 22.89,24.49 21.46,25.91
  Bottom 0.254: U1.26 2.36,30.28 | J9.6 28.09,5.44 27.28,4.62 19.15,4.62 J9.10 | v21.34,19.86 21.34,13.41 v16.87,8.94 | v4.45,26.29 4.45,28.37 U1.26 | v1.27,34.16 1.27,31.55 U1.26
VIN  (via drill 0.6)
  Top 0.406: C15.2 3.68,20.07 3.68,22.66
  Top 0.61: U1.23 3.68,22.66 5.33,22.66 10.21,17.78 v31.5,17.78 | J8.1 42.11,15.19 31.7,15.19 v31.55,15.04
  Bottom 0.61: v31.5,17.78 31.55,17.48 v31.55,15.04
VMM  (via drill 0.41, 0.6)  (1 unrouted)
  Top 0.254: C1.2 6.35,38.48 v6.22,38.35 | 17.27,42.29 17.4,42.42 19.3,42.42 20.57,41.15 20.57,38.1 20.7,37.97 C6.2 | C8.2 34.8,38.86 34.42,39.24 34.42,41.78 33.78,42.42 v31.24,42.42 | C12.+ 21.08,55.75 21.59,56.26 | IC1.22 15.2,43.27 v15.49,43.56 | IC2.22 28.92,42.89 v29.59,43.56 | IC3.22 43.14,43.14 v43.69,43.69
  Top 0.305: IC1.28 12.2,43.17 v11.81,43.56 | IC2.28 25.92,43.17 v25.53,43.56 | IC3.28 40.14,43.3 v39.75,43.69 | 5.59,56.13 5.59,55.24 C10.+
  Top 0.61: v19.43,55.12 C12.+ v22.73,55.12 | v22.73,56.39 21.72,56.39 21.59,56.26 | v19.43,56.39 21.08,56.39 | v34.44,56.39 v31.29,56.39 | C13.+ v34.49,55.17 v31.29,55.07
  Top 1.016: J4.2 6.1,59.94 5.59,59.44 5.59,56.64 | 5.46,55.12 C10.+ | 5.59,56.64 5.59,56.13 | C11.2 5.33,56.9 5.59,56.64
  Bottom 0.254: v11.81,43.56 9.65,43.56 6.22,40.13 v6.22,38.35
  Bottom 0.305: v39.75,43.69 32.51,43.69 v31.24,42.42 | v25.53,43.56 v15.49,43.56 v11.81,43.56
  Bottom 1.016: J8.2 44.96,13.97 44.96,12.6 43.56,11.2 43.56,8.13 J16.2 43.56,6.99 J17.2
  other vias: 17.27,42.42 5.33,41.4 5.08,33.91 43.28,56.39 43.28,54.36 46.33,56.44 46.38,54.46
  pour Bottom (isolate 0.406): 4.95,40.13 10.16,40.13 10.03,42.67 16.26,42.67 16.26,41.53 24.89,41.53 24.89,42.67 29.84,42.67 29.84,41.53 39.24,41.53 39.24,42.8 44.2,42.8 44.2,41.53 47.24,41.53 47.24,44.83 9.91,44.83 9.91,60.83 8.64,60.83 8.64,68.45 4.83,68.45
  pour Bottom (isolate 0.406): 9.65,57.02 47.27,57.12 47.27,54.33 9.65,54.23
  pour Bottom: 44.45,0 44.45,8.64 9.78,8.25 9.65,35.18 4.57,35.18 4.57,-0.25
  pour Top: 4.47,41.83 6.07,41.78 5.97,33.15 4.45,33.15
  pour Top: 42.47,56.95 46.99,56.95 46.99,53.9 42.47,53.9
  pour Bottom: 46.58,41.5 48.67,41.5 48.67,57.3 46.58,57.3

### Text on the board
tPlace: Power | - | + | 2B | 2A | 1A | 1B | 2B | 2A | 1A | 1B | 2B | 2A | 1A | 1B | A | B | C | 13 | 10 | I | A | I | B | I | C | MS1-3 | MS1-3 | MS1-3 | ON | A | ON | B | ON | C | GND | GND | GND | 3-StepperMotor M-Shield | Arduino Pins to Driver-IC | PWR to Arduino | D2 | D3 | D4 | D5 | D7 | D6 | DIR | STEP | DIR | STEP | DIR | STEP | Power | D8 | D9 | D12 | D10 | D13 | D11 | + | - | A | B | C | Control | Port | 8-35V
bPlace: 8-35V | Max Output: 35V/2A | - | + | 3-StepperMotor M-Shield | POWER | 2016-03-02 | www.NOA-Labs.com | Configuration: | Potentiometer: PWM Current Limitation | MAX | MIN | Triple-Switch: Microstep | Microstep Resolution | MS3 | MS2 | MS1 | 1 (Full Step) | L | L | L | 2 (Half Step) | L | L | H | 4 (Quarter Step) | L | H | L | 8 (Eighth Step) | L | H | H | 16 (Sixteenth Step) | H | H | H | POWER | - | + | A | B | C | DIR: | 5V/3V3 | 5V/3V3 | GND | GND | 8-35V | A | B | C | STEP:
tNames: J15 | J7 | J5 | J6 | J4 | J3 | J2 | J1 | C14 | D1 | J10 | J12 | J11 | J18 | J20 | J22 | J8 | J13 | J16 | J9 | J17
